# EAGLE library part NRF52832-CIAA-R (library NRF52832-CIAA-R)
Multi Protocal Bluetooth Smart ANT 2.4GHz RF SoC (WL-CSP)
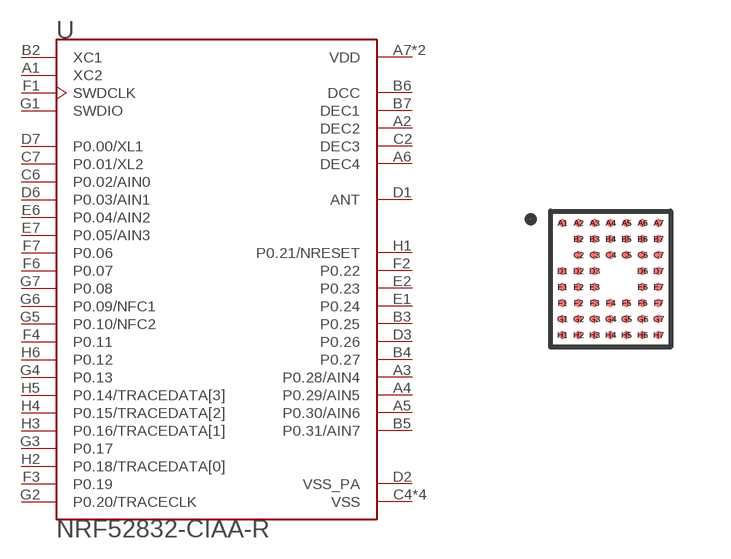
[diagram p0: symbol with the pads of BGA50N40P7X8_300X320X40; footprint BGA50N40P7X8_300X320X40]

Designator prefix U

## NRF52832-CIAA-R (AVAILABILITY: Good; DESCRIPTION: IC RF TXRX+MCU BLUETOOTH 50WLCSP; MF: Nordic; MP: NRF52832-CIAA-R; PACKAGE: XFBGA-50 Nordic Semiconductor; PRICE: 3.87 USD)  [BGA50N40P7X8_300X320X40]
A1  XC2  in
A2  DEC2  pwr
A3  P0.28/AIN4
A4  P0.29/AIN5
A5  P0.30/AIN6
A6  DEC4  pwr
A7  VDD  pwr
B2  XC1  in
B3  P0.25
B4  P0.27
B5  P0.31/AIN7
B6  DCC  pwr
B7  DEC1  pwr
C2  DEC3  pwr
C4  VSS  pwr
C5  VSS  pwr
C6  P0.02/AIN0
C7  P0.01/XL2
D1  ANT  pas
D2  VSS_PA  pwr
D3  P0.26
D6  P0.03/AIN1
D7  P0.00/XL1
E1  P0.24
E2  P0.23
E3  VSS  pwr
E6  P0.04/AIN2
E7  P0.05/AIN3
F1  SWDCLK  in
F2  P0.22
F3  P0.19
F4  P0.11
F5  VSS  pwr
F6  P0.07
F7  P0.06
G1  SWDIO
G2  P0.20/TRACECLK
G3  P0.17
G4  P0.13
G5  P0.10/NFC2
G6  P0.09/NFC1
G7  P0.08
H1  P0.21/NRESET
H2  P0.18/TRACEDATA[0]
H3  P0.16/TRACEDATA[1]
H4  P0.15/TRACEDATA[2]
H5  P0.14/TRACEDATA[3]
H6  P0.12
H7  VDD  pwr

## Footprint BGA50N40P7X8_300X320X40 (pad centres in mm)
smd 0.2 x 0.2: A1 -1.2,1.4; A2 -0.8,1.4; A3 -0.4,1.4; A4 0,1.4; A5 0.4,1.4; A6 0.8,1.4; A7 1.2,1.4; B2 -0.8,1; B3 -0.4,1; B4 0,1; B5 0.4,1; B6 0.8,1; B7 1.2,1; C2 -0.8,0.6; C3 -0.4,0.6; C4 0,0.6; C5 0.4,0.6; C6 0.8,0.6; C7 1.2,0.6; D1 -1.2,0.2; D2 -0.8,0.2; D3 -0.4,0.2; D6 0.8,0.2; D7 1.2,0.2; E1 -1.2,-0.2; E2 -0.8,-0.2; E3 -0.4,-0.2; E6 0.8,-0.2; E7 1.2,-0.2; F1 -1.2,-0.6; F2 -0.8,-0.6; F3 -0.4,-0.6; F4 0,-0.6; F5 0.4,-0.6; F6 0.8,-0.6; F7 1.2,-0.6; G1 -1.2,-1; G2 -0.8,-1; G3 -0.4,-1; G4 0,-1; G5 0.4,-1; G6 0.8,-1; G7 1.2,-1; H1 -1.2,-1.4; H2 -0.8,-1.4; H3 -0.4,-1.4; H4 0,-1.4; H5 0.4,-1.4; H6 0.8,-1.4; H7 1.2,-1.4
